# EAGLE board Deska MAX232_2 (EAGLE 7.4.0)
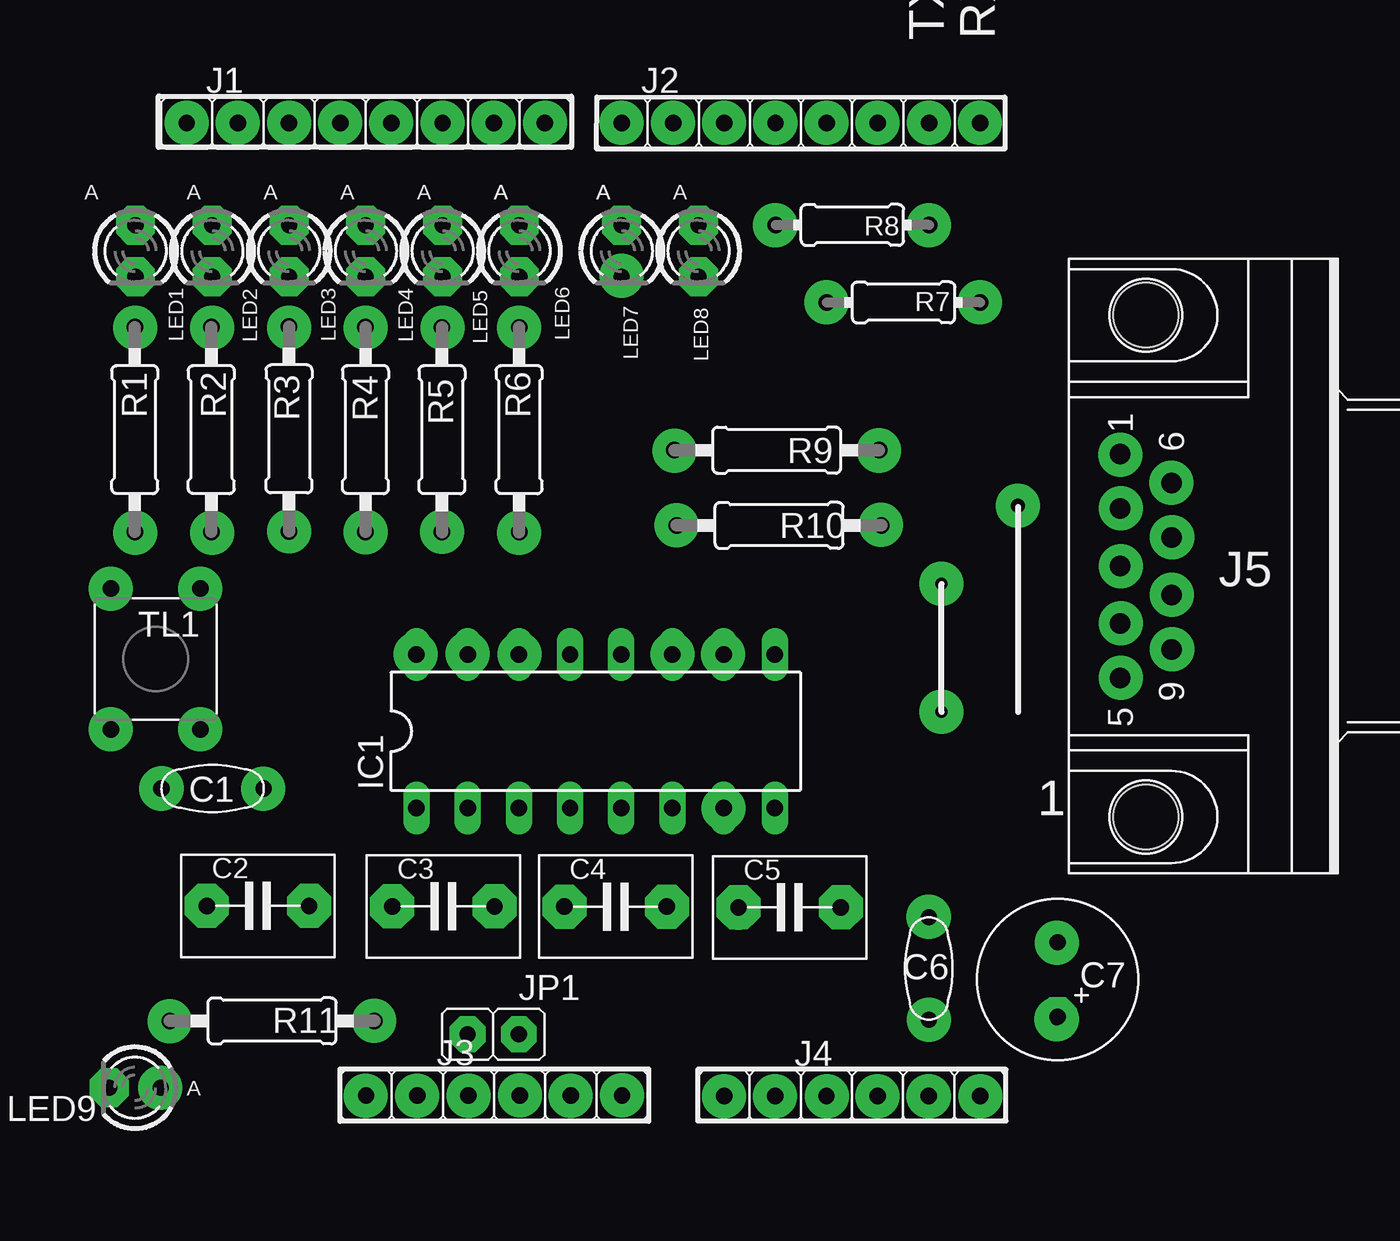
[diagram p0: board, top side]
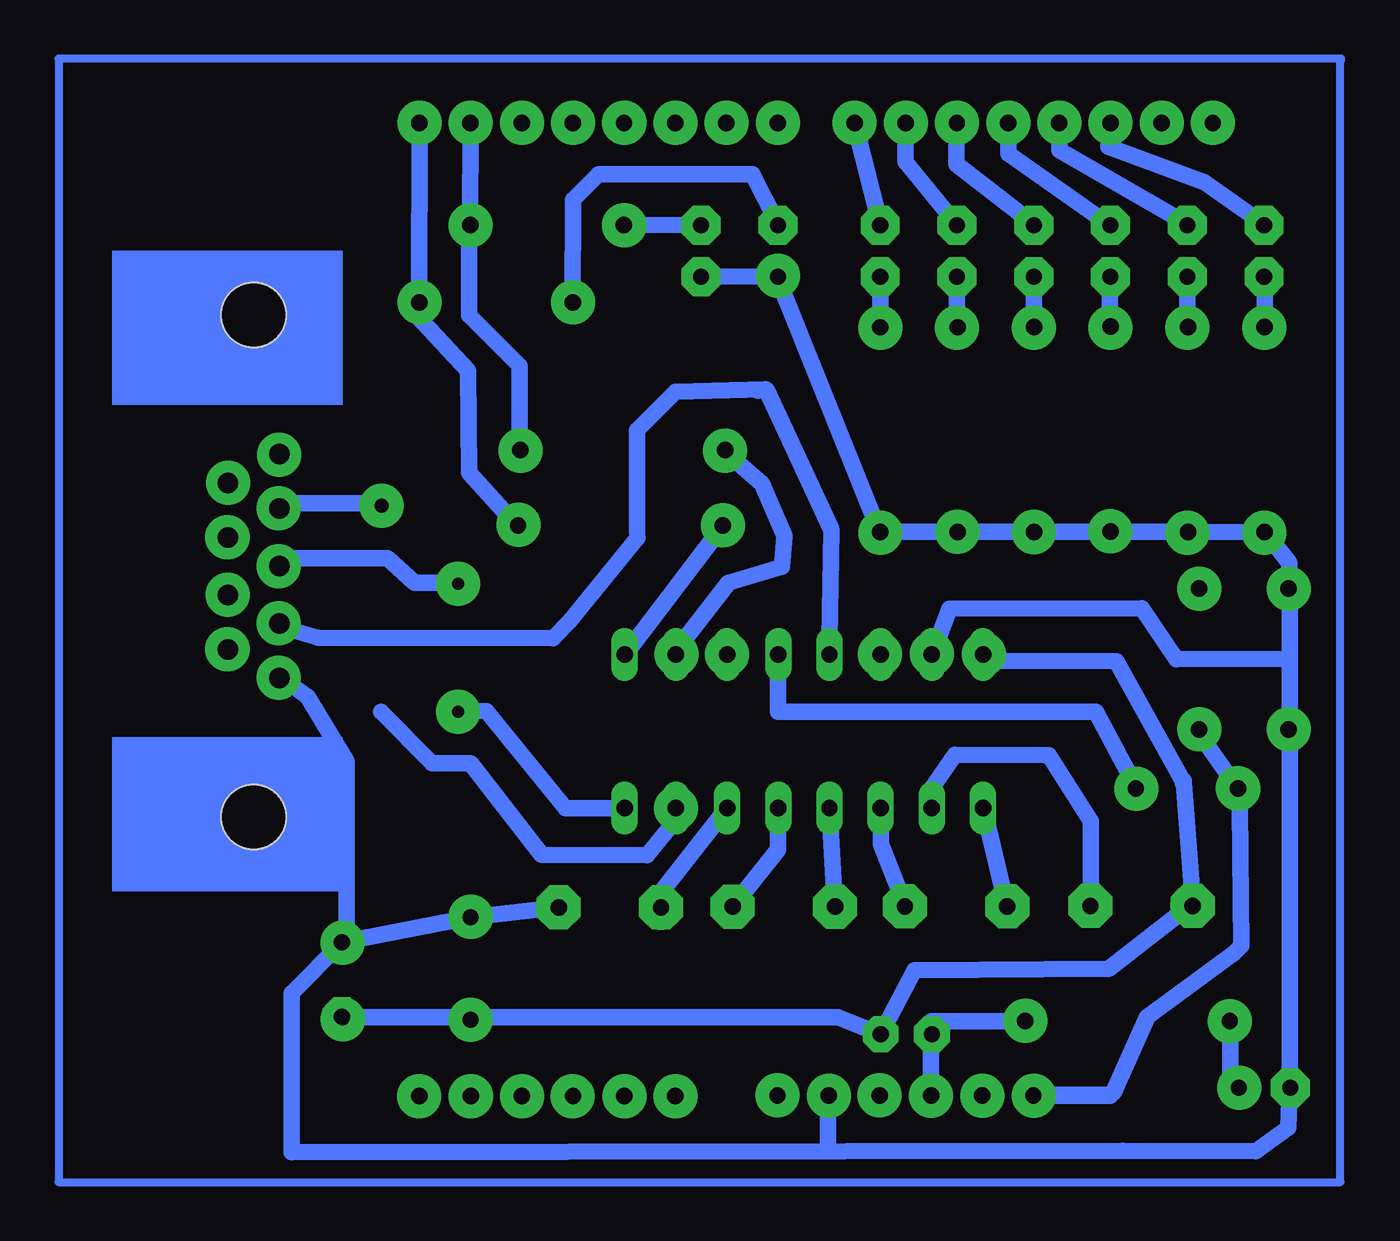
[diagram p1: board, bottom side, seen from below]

No outline drawn. Coordinates in mm, seen from the top.
Copper layers (1*16): Top 0.035mm / dielectric 1.5mm / Bottom 0.035mm
Design rules "default": minimum track width 6mil, minimum drill 0.35mm, track to track 6mil, track to pad 6mil, pad to pad 6mil, via to via 6mil, smd to smd 6mil, copper to edge 40mil, drill to drill 6mil, minimum pad ring 10mil, minimum via ring 8mil, stop-mask expansion 4mil, vias tented up to drill 0mil, thermal gap 10mil

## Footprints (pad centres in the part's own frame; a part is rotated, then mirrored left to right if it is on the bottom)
KERAMICKY_RM5 = drill 0.8 pad 1.93 octagon: P$1 -2.54,0; P$2 2.54,0
RM5_5,0 = drill 0.813 pad 2.184 octagon: 1 -2.54,0; 2 2.54,0
ELEKTROLITICKY_RM3,5-8 = drill 0.8 pad 1.93 octagon: P$1 -1.84,0; P$2 1.84,0
DIL16 = drill 0.813 long: 1 -8.89,-3.81; 2 -6.35,-3.81; 3 -3.81,-3.81; 4 -1.27,-3.81; 5 1.27,-3.81; 6 3.81,-3.81; 7 6.35,-3.81; 8 8.89,-3.81; 9 8.89,3.81; 10 6.35,3.81; 11 3.81,3.81; 12 1.27,3.81; 13 -1.27,3.81; 14 -3.81,3.81; 15 -6.35,3.81; 16 -8.89,3.81
S1G8_JUM = drill 0.813 pad 1.778 octagon: 1 -8.89,0; 2 -6.35,0; 3 -3.81,0; 4 -1.27,0; 5 1.27,0; 6 3.81,0; 7 6.35,0; 8 8.89,0
S1G6_JUM = drill 0.813 pad 1.778 octagon: 1 -6.35,0; 2 -3.81,0; 3 -1.27,0; 4 1.27,0; 5 3.81,0; 6 6.35,0
CAN9Z/90 = drill 1.016 pad 1.93 octagon: 1 -5.556,0; 2 -2.857,0; 3 0,0; 4 2.857,0; 5 5.556,0; 6 -4.128,2.54; 7 -1.429,2.54; 8 1.429,2.54; 9 4.128,2.54 | hole 3.2: 12.446,1.27; -12.446,1.27
S1G2_JUM = drill 0.813 pad 1.778 octagon: 1 -1.27,0; 2 1.27,0
LED3MM = drill 0.8 pad 1.93 octagon: A -1.27,0; K 1.27,0
0207/10 = drill 0.813 octagon: 1 -5.08,0; 2 5.08,0
0204/7 = drill 0.813 octagon: 1 -3.81,0; 2 3.81,0
P-B1720 = drill 0.813 pad 1.93 octagon: 1 -3.493,-2.223; 2 -3.493,2.223; 3 3.493,-2.223; 4 3.493,2.223

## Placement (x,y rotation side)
C1  100n  [KERAMICKY_RM5]  -137.14,26.67 180 top
C2  1u  [RM5_5,0]  -134.89,20.85 0 top
C3  1u  [RM5_5,0]  -125.69,20.82 0 top
C4  1u  [RM5_5,0]  -117.14,20.81 0 top
C5  1u  [RM5_5,0]  -108.5,20.77 0 top
C6  100n  [KERAMICKY_RM5]  -101.6,17.75 90 top
C7  47u  [ELEKTROLITICKY_RM3,5-8]  -95.21,17.2 270 top
IC1  MAX232  [DIL16]  -118.13,29.52 0 top
J1  [S1G8_JUM]  -129.54,59.69 0 top
J2  [S1G8_JUM]  -107.94,59.69 0 top
J3  [S1G6_JUM]  -123.17,11.45 0 top
J4  [S1G6_JUM]  -105.41,11.42 0 top
J5  [CAN9Z/90]  -92.1,37.71 270 top
JP1  [S1G2_JUM]  -123.22,14.49 0 top
LED1  [LED3MM]  -140.97,53.34 270 top
LED2  [LED3MM]  -137.16,53.34 270 top
LED3  [LED3MM]  -133.35,53.34 270 top
LED4  [LED3MM]  -129.54,53.34 270 top
LED5  [LED3MM]  -125.73,53.34 270 top
LED6  [LED3MM]  -121.92,53.34 270 top
LED7  [LED3MM]  -116.84,53.34 270 top
LED8  [LED3MM]  -113.03,53.34 270 top
LED9  [LED3MM]  -140.99,11.83 180 top
R1  1k  [0207/10]  -141,44.48 90 top
R2  1k  [0207/10]  -137.2,44.48 90 top
R3  1k  [0207/10]  -133.35,44.51 90 top
R4  1k  [0207/10]  -129.55,44.48 90 top
R5  1k  [0207/10]  -125.76,44.47 90 top
R6  1k  [0207/10]  -121.93,44.48 90 top
R7  1k  [0204/7]  -102.85,50.79 0 top
R8  1k  [0204/7]  -105.39,54.63 0 top
R9  1k  [0207/10]  -109.15,43.46 0 top
R10  1k  [0207/10]  -109.03,39.73 0 top
R11  1k  [0207/10]  -134.19,15.14 0 top
TL1  [P-B1720]  -139.96,33.1 270 top

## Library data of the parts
C1 C6 C7 = #Kondenzatory
C2-C5 = #PaJa_C-folie
IC1 = 41xx
J1-J5 JP1 = #PaJa_konektory
LED1-LED9 = #Led
R1-R11 = resistor
TL1 = #PaJa_prepinace

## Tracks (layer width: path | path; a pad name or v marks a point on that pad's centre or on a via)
S$1  (via drill 0.6 pad 2.18)
  other vias: -101.6,11.42 -101.6,20.31 -95.25,15.23
S$2
  Bottom 0.813: -110.96,21.44 -114.32,25.69
S$3  (via drill 0.6 pad 2.18)
  other vias: -126.99,11.44 -124.45,11.44
S$4
  Bottom 0.813: -133.32,54.62 -128.28,58.16 -128.27,59.69
S$5  (via drill 0.6 pad 2.18)
  other vias: -121.89,11.45
S$6  (via drill 0.6 pad 2.18)
  Bottom 0.813: v-129.54,11.43 -133.35,11.43
S$7  (via drill 0.6 pad 2.18)
  other vias: -116.82,11.45
S$8
  Bottom 0.813: -128.21,20.81 -127.03,25.71
S$9  (via drill 0.6 pad 2.18)
  other vias: -111.76,11.4 -101.6,15.21
S$10  (via drill 0.6 pad 2.18)
  other vias: -109.23,11.41
S$11  (via drill 0.6 pad 2.18)
  other vias: -104.15,11.41
S$12
  Bottom 0.813: -124.45,11.44 -124.44,15.11
S$13  (via drill 0.6 pad 2.18)
  other vias: -106.66,11.41
S$14  (via drill 0.6 pad 2.18)
  other vias: -121.91,33.33
S$15
  Bottom 0.813: -123.16,20.83 -121.96,23.9 -121.96,25.73
S$16
  Bottom 0.813: -121.94,14.49 -119.83,15.33 -95.2,15.32
S$17
  Bottom 0.813: -137.18,54.67 -130.81,58.34 -130.81,59.69
S$18  (via drill 0.6 pad 2.18)
  Bottom 0.813: -137.17,52.09 v-137.16,49.53
S$19
  Bottom 0.813: -116.84,54.66 -115.57,57.15 -107.95,57.15 -106.68,55.88 -106.66,50.79
S$20
  Bottom 0.813: -113.06,54.62 -109.2,54.64
S$21  (via drill 0.6 pad 2.18)
  other vias: -116.84,59.69
S$22  (via drill 0.6 pad 2.18)
  other vias: -114.3,59.69
S$23  (via drill 0.6 pad 2.18)
  other vias: -111.76,59.69
S$24
  Bottom 0.813: -109.86,39.12 -106.54,34.99 -105.69,34.13 -94.02,34.15 -91.89,34.77
S$25
  Bottom 0.813: -141.01,54.65 -138,56.74 -133.25,58.52 -133.35,59.69
S$26
  Bottom 0.813: -129.11,15.12 -124.47,15.12
S$27  (via drill 0.6 pad 2.18)
  other vias: -119.38,11.43
S$28
  Bottom 0.813: -119.39,11.53 -119.4,11.53
S$29  (via drill 0.6 pad 2.18)
  other vias: -138.43,59.69
S$30
  Bottom 0.813: -119.68,20.8 -119.39,25.69
S$31
  Bottom 0.813: -114.59,20.81 -116.85,23.63 -116.88,25.7
S$32
  Bottom 0.813: -119.41,11.4 -119.32,11.4 -119.32,8.69
S$33  (via drill 0.6 pad 2.18)
  other vias: -139.73,11.83
S$34
  Bottom 0.813: -139.64,11.78 -139.3,11.78 -139.3,15.17
S$35  (via drill 0.6 pad 2.18)
  other vias: -114.31,33.34
S$36  (via drill 0.6 pad 2.18)
  other vias: -111.8,33.33
S$37  (via drill 0.6 pad 2.18)
  other vias: -104.14,59.69 -101.6,59.69 -99.06,59.69
S$38  (via drill 0.6 pad 2.18)
  other vias: -99.05,11.41 -95.24,19.03
S$39
  Bottom 0.813: -137,27.06 -137,26.94 -137.45,20.81
S$40
  Bottom 0.813: -129.55,54.66 -125.7,57.65 -125.73,59.69
S$41
  Bottom 0.813: -139.7,26.69 -139.77,25.71 -139.84,18.86 -139.47,18.49 -135.19,15.36 -133.5,11.58
S$42
  Bottom 0.813: -125.72,54.64 -123.18,57.77 -123.19,59.69
S$43  (via drill 0.6 pad 2.18)
  other vias: -116.85,52.11
S$44
  Bottom 0.813: -121.92,54.61 -120.65,59.69
S$45  (via drill 0.6 pad 2.18)
  Bottom 0.813: -141.02,52.11 v-140.97,49.53
S$46
  Bottom 0.813: -132.35,20.84 -132.38,21.08 -132.38,25.05 -130.28,28.32 -125.63,28.34 -124.46,26.67 -124.48,25.7
S$47
  Bottom 0.813: -133.31,52.08 -133.31,49.54
S$48  (via drill 0.6 pad 2.18)
  Bottom 0.813: -129.55,52.1 v-129.54,49.53
S$49
  Bottom 0.813: -101.57,54.64 -101.6,59.69
S$50  (via drill 0.6 pad 2.18)
  Bottom 0.813: -125.73,52.07 v-125.73,49.53
S$51
  Bottom 0.813: -109.22,33.29 -114.13,39.71
S$52  (via drill 0.6 pad 2.18)
  Bottom 0.813: -121.92,52.07 v-121.92,49.53
S$53  (via drill 0.6 pad 2.18)
  other vias: -111.05,20.76
S$54  (via drill 0.6 pad 2.18)
  other vias: -139.68,26.68
S$55
  Bottom 0.813: -137.31,20.87 -133.27,17.73 -123.63,17.67 -121.89,14.37
S$56
  Bottom 0.813: -139.67,26.67 -137.63,29.56
S$57  (via drill 0.6 pad 2.18)
  other vias: -127.06,33.33
S$58  (via drill 0.6 pad 2.18)
  other vias: -133.34,39.43
S$59  (via drill 0.6 pad 2.18)
  other vias: -124.49,33.37
S$60  (via drill 0.6 pad 2.18)
  other vias: -135.89,59.69 -133.35,59.69 -130.81,59.69 -128.27,59.69 -125.73,59.69 -123.19,59.69 -120.65,59.69
S$61  (via drill 0.6 pad 2.18)
  other vias: -129.55,39.4
S$62  (via drill 0.6 pad 2.18)
  other vias: -109.22,59.69
S$63  (via drill 0.6 pad 2.18)
  other vias: -106.68,59.69
S$64  (via drill 0.6 pad 2.18)
  other vias: -125.76,39.41
S$65
  Bottom 0.813: -113.02,52.09 -116.84,52.07 -116.84,51.93 -121.83,39.52 -121.92,39.43 -121.94,39.41 -137.2,39.41 -141.03,39.38 -142.23,37.88 -142.24,35.56 -142.24,21.02 -142.24,11.81 -142.17,9.86 -140.56,8.67 -133.97,8.7 -92.71,8.63 -92.71,16.51 -95.22,19.04 -101.58,20.29 -105.98,20.77
S$66
  Bottom 0.813: -111.9,25.28 -110.35,23.36 -105.11,23.4 -101.6,27.94 -99.69,27.94 -97.16,30.48
S$67
  Bottom 0.813: -99.05,50.78 -99.06,59.69
S$68
  Bottom 0.813: -109.24,25.69 -106.32,25.69 -102.38,30.51 -100.51,30.55
S$69
  Bottom 0.813: -126.98,33.01 -133.63,32.98 -137,26.96 -136.94,26.93
S$70
  Bottom 0.813: -124.52,33.32 -125.35,35.59 -134.91,35.61 -136.62,33.08 -142.18,33.1
S$72
  Bottom 0.813: -129.44,11.47 -133.26,11.52
S$73  (via drill 0.6 pad 2.18)
  other vias: -111.8,25.69
S$74  (via drill 0.6 pad 2.18)
  other vias: -129.13,15.15 -129.13,15.15 -137.75,29.61 -142.19,29.61 -142.19,36.58 -137.75,36.59 -137.42,20.85
S$75  (via drill 0.6 pad 2.18)
  other vias: -139.28,15.12
S$76
  Bottom 0.813: -92.24,32.15 -93.51,31.23 -95.44,28.03 -95.44,19.15 -95.36,19.08
S$77  (via drill 0.6 pad 2.18)
  other vias: -114.21,43.43
S$78
  Bottom 0.813: -111.77,33.55 -111.72,33.46 -114.39,36.88 -117.03,37.68 -117.17,39.21 -116.05,41.8 -114.14,43.46
S$79  (via drill 0.6 pad 2.18)
  other vias: -103.97,39.76
S$80
  Bottom 0.813: -98.92,50.83 -98.92,50.16 -101.48,47.4 -101.52,42.33 -103.95,39.65
S$81  (via drill 0.6 pad 2.18)
  other vias: -104.07,43.44
S$82
  Bottom 0.813: -116.84,33.29 -116.84,30.48 -132.63,30.47 -134.63,26.7 -134.63,26.68
S$83
  Bottom 0.813: -101.52,54.64 -101.52,50.16 -104.03,47.65 -104.03,43.55 -103.99,43.51
S$84
  Bottom 0.813: -119.44,33.27 -119.39,34.08 -119.49,39.51 -116.27,46.45 -115.85,46.41
S$85
  Bottom 0.813: -97.15,40.82 -92.24,40.82 -92.1,40.67
S$86  (via drill 0.6 pad 2.18)
  other vias: -100.97,30.48
S$87
  Bottom 0.813: -97.31,38.11 -92.08,38.1
S$88
  Bottom 0.813: -116.22,46.47 -111.76,46.35 -109.86,44.45 -109.86,39.37
S$89  (via drill 0.7 pad 2.18)
  other vias: -92.1,43.24
S$90  (via drill 0.7 pad 2.18)
  other vias: -89.56,41.84
S$91  (via drill 0.7 pad 2.18)
  other vias: -92.08,40.57
S$92  (via drill 0.7 pad 2.18)
  other vias: -89.52,39.14
S$93  (via drill 0.7 pad 2.18)
  other vias: -92.06,37.69
S$94  (via drill 0.7 pad 2.18)
  other vias: -89.54,36.28
S$95  (via drill 0.7 pad 2.18)
  other vias: -92.06,34.87
S$96  (via drill 0.7 pad 2.18)
  other vias: -89.52,33.58
S$97  (via drill 0.7 pad 2.18)
  other vias: -92.08,32.16
S$98  (via drill 0.7 pad 2.18)
  other vias: -90.87,25.27
S$99  (via drill 0.7 pad 2.18)
  other vias: -90.84,50.11
S$100  (via drill 0.7 pad 2.18)
  other vias: -97.18,40.7
S$101  (via drill 0.6 pad 2.18)
  other vias: -100.97,36.83
S$102
  Bottom 0.813: -101.04,36.89 -98.81,36.89 -97.48,38.1
S$103
  Bottom 0.406: -144.78,62.8 -144.78,62.88 -81.15,62.88 -81.15,7.15 -144.76,7.15 -144.76,62.87 -144.72,62.87
S$104  (via drill 0.6 pad 2.18)
  other vias: -140.97,39.37
S$105  (via drill 0.6 pad 2.18)
  other vias: -137.16,39.37
S$106  (via drill 0.6 pad 2.18)
  other vias: -121.92,39.37
S$107  (via drill 0.6 pad 2.18)
  other vias: -133.35,49.53
S$108  (via drill 0.6 pad 2.18)
  other vias: -106.68,50.8
S$109  (via drill 0.6 pad 2.18)
  other vias: -109.22,54.61
S$110  (via drill 0.6 pad 2.18)
  other vias: -101.6,54.61
S$111  (via drill 0.6 pad 2.18)
  other vias: -99.06,50.8
S$112  (via drill 0.6 pad 2.18)
  other vias: -134.62,26.67
S$113  (via drill 0.6 pad 2.18)
  other vias: -139.7,26.67
S$115  (via drill 0.6 pad 2.18)
  other vias: -114.11,39.73
(copper drawn outside any net)
  shapes: Bottom area x2

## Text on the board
tPlace: TX | RX | A | A | A | A | A | A | A | A | A | A | 1 | A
